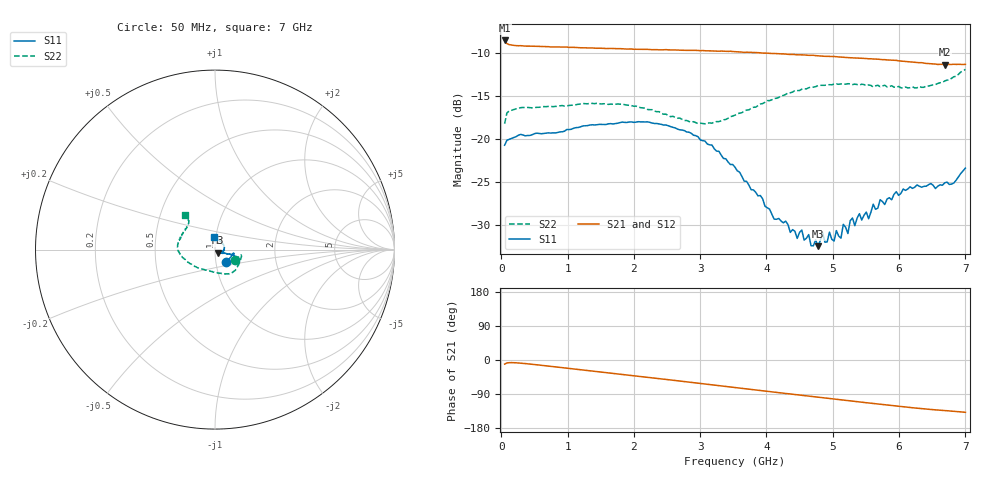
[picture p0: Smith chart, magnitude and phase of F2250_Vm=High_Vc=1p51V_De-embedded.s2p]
! Integrated Device Technology
! Corporate Headquarters
! 6024 Silver Creek Valley Road
! San Jose, CA 95138  USA
! Phone:  1-408-284-8200
! Toll Free:  1-800-223-1366
! Webpage:  http://www.idt.com/
! Timing and RF Division
! 515 Groton Road, Suite 102
! Westford, MA 01886-6024
! Device:  F2250
! Description: Voltage Variable RF Attenuator
! Frequency:  50.0 -  6000.00 MHz
! Package:  3x3 mm Thin QFN Plastic Package: 16 pin
! Ports:  2 RF, 3 DC
!  Pin  1  = GND
!  Pin  2  = NC
!  Pin  3  = RF1  = Port 1
!  Pin  4  = NC
!  Pin  5  = GND
!  Pin  6  = GND
!  Pin  7  = GND
!  Pin  8  = GND
!  Pin  9  = NC
!  Pin 10  = RF2  = Port 2
!  Pin 11  = NC
!  Pin 12  = GND
!  Pin 13  = GND
!  Pin 14  = VCNTRL
!  Pin 15  = VDD
!  Pin 16  = VMODE
! Vcntrl:  1.510 Volts
! Vmode:  +3.300 Volts
! Vdd:  +3.30  Volts
! Current:  1.329 mA
! Data:  The device was measured on a the F2250 evaluation board which has
!  individual transmission lines to the RF pins.  Data was collected
!  using a calibrated network analyzer.  The evaluation board was
!  de-embedded using a TRL calibration technique.
!  The reference plane is the edge of the package pin.
! Misc:  SN 10
!  Action Tracker AT0258
! Date Measured:  2014-11-26
! Date:  2015-10-15  MJV
! Note:
!  Integrated Device Technology supplies this data as a sample of measured
!  data at the package pin for this product.  Your particular data for this
!  product may vary.
!  Data was taken at 25 degrees C.
!  Integrated Device Technology reserves the right to change this data at anytime.
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# GHz S dB R 50
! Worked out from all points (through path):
!   201 points, 50 MHz to 7 GHz, reference 50 ohm
!   highest |S21| = -8.49 dB at 50 MHz (marker M1); lowest = -11.3 dB at 6.687 GHz (marker M2)
!   group delay of S21, straight-line fit = 55.1 ps
!   lowest |S11| = -32.5 dB at 4.776 GHz (marker M3), VSWR 1.05, Z = 51.6 - j1.82 ohm
!   |S11| at or under -10 dB: start of sweep to end of sweep
!   |S22| runs from -18.2 to -11.9 dB; largest |S21 - S12| = 0.0017
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0.05  -20.73 -46.8  -8.49 -10.8  -8.48 -10.7  -18.22 -27.7
0.08475  -20.15 -24.3  -8.86 -7.9  -8.88 -7.9  -16.95 -15.2
0.29325  -19.47 -10.9  -9.10 -8.3  -9.14 -8.3  -16.34 -14.1
1.2315  -18.48 -21.5  -9.35 -26.4  -9.34 -26.4  -15.87 -42.3
2.37825  -18.24 -19.6  -9.59 -49.1  -9.59 -49.1  -16.81 -70.4
2.969  -19.75 -16.3  -9.67 -61.2  -9.67 -61.2  -18.21 -98.0
3.525  -23.30 -19.1  -9.80 -72.7  -9.82 -72.7  -17.22 -132.2
4.11575  -29.36 -32.8  -10.02 -84.8  -10.00 -84.9  -15.26 -158.9
4.7065  -32.48 -52.2  -10.23 -96.9  -10.25 -96.8  -13.95 -175.7
4.776  -32.52 -48.2  -10.29 -98.2  -10.30 -98.2  -13.77 -177.5
4.8455  -30.93 -48.3  -10.31 -99.6  -10.31 -99.6  -13.74 -178.7
4.88025  -32.05 -43.0  -10.35 -100.3  -10.36 -100.3  -13.73 -180.0
4.94975  -30.88 -46.7  -10.36 -101.7  -10.34 -101.8  -13.66 178.5
5.1235  -31.59 -46.9  -10.43 -105.2  -10.44 -105.2  -13.57 174.2
5.15825  -29.98 -44.2  -10.46 -105.8  -10.46 -105.9  -13.55 173.8
5.22775  -31.04 -38.5  -10.49 -107.2  -10.49 -107.3  -13.54 171.9
5.29725  -29.23 -30.0  -10.53 -108.5  -10.55 -108.5  -13.65 170.5
5.5405  -29.32 -21.7  -10.64 -113.4  -10.63 -113.5  -13.69 163.8
5.61  -27.62 -21.6  -10.66 -114.7  -10.65 -114.8  -13.92 162.5
5.85325  -26.86 -11.9  -10.78 -119.4  -10.79 -119.6  -13.89 155.2
6.68725  -25.14 49.0  -11.31 -133.4  -11.31 -133.6  -13.23 132.0
7  -23.40 92.4  -11.28 -138.0  -11.27 -138.2  -11.87 131.7
